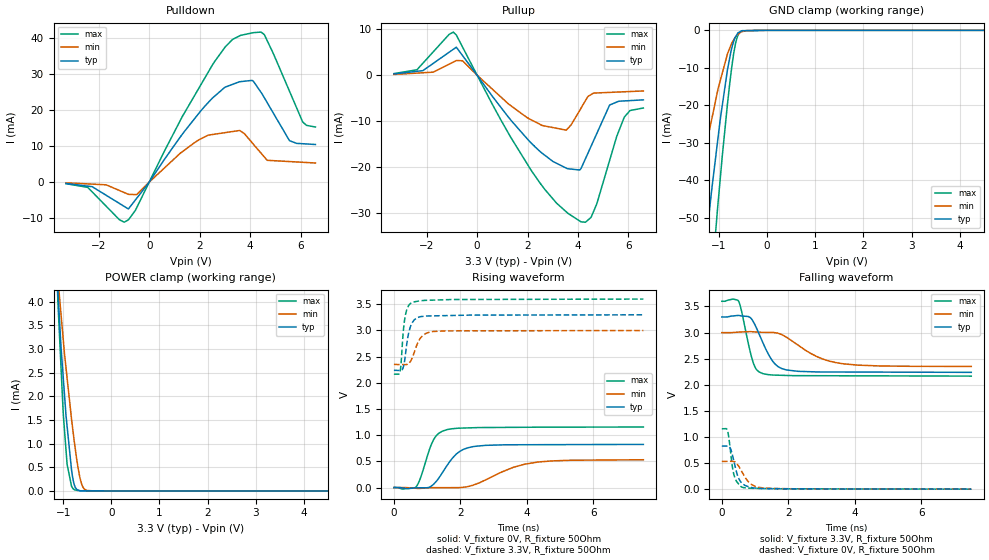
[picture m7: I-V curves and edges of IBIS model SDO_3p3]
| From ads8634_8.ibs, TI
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|   SDO_3p3  3.3V digital 3-state Model
[Model] SDO_3p3  | 3.3V digital 3-state
Model_type 3-state
Polarity   Non-Inverting
Vmeas = 1.65
Vref = 1.65
Cref = 15pF
Rref = 50
|   typ   min   max
|   (nom PVT)   (Fast PVT)   (slow PVT)
|BUFFER OUTPUT TURNED HIGH
|C_comp from L-C Tank method(L=1nH)
|Resonant Frequency(Hz)   4.38G   4.81G   3.96G
|C_comp   1.32459E-12   1.09668E-12   1.61466E-12
|BUFFER OUTPUT LOW
|C_comp from L-C Tank method(L=1nH)
|Resonant Frequency(Hz)   4.29G   4.70G   3.95G
|C_comp   1.38064E-12   1.14552E-12   1.62211E-12
|BUFFER HIGH Z STATE
|C_comp from L-C Tank method(L=1nH)
|Resonant Frequency(Hz)   4.04G   4.41G   3.82G
C_comp   1.55626E-12   1.30641E-12   1.73813E-12
| Where   nom PVT is  Nominal Process, 3.3V, 25C
|   Fast PVT is Strong Process, 3.6V, -40C
|   Slow PVT is Weak Process, 3.0V, 85C
|C_comp - from L-C Tank method, L = 1nH, peak frequency
[Voltage Range]   3.3   3   3.6
[Temperature Range]   27   125   -40
[Pullup Reference]   3.3   3   3.6
[Pulldown Reference]   0   0   0
[Power Clamp Reference]   3.3   3   3.6
[GND Clamp Reference]   0   0   0
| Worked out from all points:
|   slope of the pulldown table from 0 to 0.495 V, typ, clamps not added: 95.7 ohm
|   slope of the pullup table from 0 to 0.495 V, typ, clamps not added: 131 ohm
|   GND clamp passes 1 mA (typ) near -0.62 V on its own axis
|   POWER clamp passes 1 mA (typ) near -0.88 V on its own axis
|   falling waveform, V_fixture 3.3V, R_fixture 50Ohm: 20-80 % time 490ps typ, 1.06ns min, 304ps max; typ from 3.3 V to 2.24 V
|   rising waveform, V_fixture 0V, R_fixture 50Ohm: 20-80 % time 585ps typ, 1.19ns min, 379ps max; typ from 0.002 V to 0.825 V
|   rising waveform, V_fixture 3.3V, R_fixture 50Ohm: 20-80 % time 178ps typ, 264ps min, 129ps max; typ from 2.24 V to 3.3 V
|   falling waveform, V_fixture 0V, R_fixture 50Ohm: 20-80 % time 225ps typ, 337ps min, 161ps max; typ from 0.825 V to 0.002 V
[Pulldown]
|   Voltage   I(typ)   I(min)   I(max)
-3.3V     -389.4uA   -204.7uA   -455.8uA
-2.443V   -1.123mA   -506.1uA   -1.449mA
-1.18V    -5.928mA   -2.343mA   -10.44mA
-825.7mV  -7.447mA   -3.402mA   -10.47mA
-499.9mV  -4.521mA   -3.471mA   -7.151mA
2.512V    23.31mA    13.18mA    32.52mA
3.623V    27.83mA    14.13mA    40.65mA
4.119V    27.98mA    10.56mA    41.38mA
4.56V     23.41mA    6.987mA    40.87mA
5.563V    11.46mA    5.681mA    25.14mA
6.088V    10.62mA    5.477mA    16.62mA
6.59V     10.41mA    5.281mA    15.26mA
[GND Clamp]
|   Voltage   I(typ)   I(min)   I(max)
-3.3V     -333.7mA   -218.9mA   -423.9mA
-1.593V   -96.69mA   -55.56mA   -138.7mA
-1.503V   -85.34mA   -48.26mA   -123.7mA
-1.25V    -54.2mA    -29.86mA   -82.25mA
-1.149V   -42.23mA   -23.57mA   -66.22mA
-1.037V   -30.41mA   -16.66mA   -48.58mA
-826mV    -10.66mA   -6.382mA   -19.88mA
-750.7mV  -5.602mA   -3.917mA   -11.44mA
-698.7mV  -3.129mA   -2.654mA   -6.526mA
-629.4mV  -1.183mA   -1.372mA   -2.157mA
-517.4mV  -87.12uA   -359.9uA   -137.8uA
6.59V     0A         0A         0A
[Pullup]
|   Voltage   I(typ)   I(min)   I(max)
-3.3V     282.6uA    176.9uA    359.9uA
-2.384V   863.4uA    472.2uA    1.213mA
-946.1mV  5.666mA    2.884mA    9.428mA
-576.3mV  4.279mA    3.161mA    6.135mA
1.311V    -9.614mA   -6.549mA   -13.35mA
2.584V    -17.05mA   -10.97mA   -24.2mA
3.534V    -20.28mA   -11.98mA   -29.82mA
4.12V     -20.32mA   -7.166mA   -32.01mA
4.518V    -15.48mA   -4.214mA   -31.01mA
5.251V    -6.512mA   -3.741mA   -18.62mA
5.834V    -5.602mA   -3.604mA   -9.139mA
6.59V     -5.371mA   -3.425mA   -7.146mA
[POWER Clamp]
|   Voltage   I(typ)   I(min)   I(max)
-3.3V     52.32mA    41.51mA    66.09mA
-1.162V   5.162mA    5.3mA      5.365mA
-1.103V   4.107mA    4.473mA    3.873mA
-1.077V   3.627mA    4.11mA     3.306mA
-1.002V   2.452mA    3.25mA     1.719mA
-918.3mV  1.371mA    2.39mA     566.7uA
-826mV    443.1uA    1.521mA    98.85uA
-762mV    112uA      993.2uA    20.84uA
-645.7mV  3.761uA    253.7uA    927.2nA
-584.5mV  2.735uA    71.72uA    604.3nA
-505.2mV  2.351uA    8.775uA    519.3nA
6.59V     0A         0A         0A
[Ramp]
R_load = 50
|   typ   min   max
dV/dt_r   0.493896/5.81927e-010  0.318267/1.16625e-009  0.693599/3.77324e-010
dV/dt_f   0.636389/4.88374e-010  0.388684/1.04617e-009  0.860088/3.02558e-010
[Falling Waveform]
V_fixture = 3.3V
V_fixture_min = 3V
V_fixture_max = 3.6V
R_fixture = 50Ohm
C_fixture = 0F
|   Time   V(typ)   V(min)   V(max)
0s        3.299V     2.999V     3.6V
504.1ps   3.328V     3.01V      3.601V
939.8ps   3.215V     3.015V     2.432V
1.053ns   3.072V     3.01V      2.283V
1.229ns   2.813V     3.005V     2.215V
1.595ns   2.401V     2.998V     2.185V
1.953ns   2.284V     2.908V     2.179V
2.849ns   2.247V     2.543V     2.174V
3.627ns   2.245V     2.404V     2.173V
7.5ns     2.238V     2.351V     2.166V
[Rising Waveform]
V_fixture = 0V
V_fixture_min = 0V
V_fixture_max = 0V
R_fixture = 50Ohm
C_fixture = 0F
|   Time   V(typ)   V(min)   V(max)
0s        1.562mV    1.115mV    646.9uV
667.2ps   -4.062mV   -13.43mV   15mV
798.6ps   -3.843mV   -14.61mV   183mV
1.185ns   58.39mV    -1.454mV   905mV
1.587ns   412.7mV    -1.243mV   1.105V
1.98ns    690.7mV    -304.9uV   1.135V
2.42ns    786.2mV    55.37mV    1.144V
3.575ns   817.7mV    383.1mV    1.15V
4.328ns   819mV      487.4mV    1.153V
7.5ns     824.7mV    531.6mV    1.157V
[Rising Waveform]
V_fixture = 3.3V
V_fixture_min = 3V
V_fixture_max = 3.6V
R_fixture = 50Ohm
C_fixture = 0F
|   Time   V(typ)   V(min)   V(max)
0s        2.238V     2.351V     2.166V
183.3ps   2.237V     2.349V     2.207V
269.2ps   2.275V     2.348V     2.883V
325.5ps   2.442V     2.348V     3.218V
384.4ps   2.733V     2.351V     3.391V
488.1ps   3.058V     2.402V     3.511V
578.3ps   3.174V     2.523V     3.543V
809.1ps   3.265V     2.864V     3.568V
1.181ns   3.279V     2.981V     3.58V
7.5ns     3.299V     2.999V     3.6V
[Falling Waveform]
|Gnd
V_fixture = 0V
V_fixture_min = 0V
V_fixture_max = 0V
R_fixture = 50Ohm
C_fixture = 0F
|   Time   V(typ)   V(min)   V(max)
0s        824.8mV    532.1mV    1.157V
167.1ps   826.4mV    533.3mV    1.128V
253.3ps   788.7mV    533.8mV    766.3mV
316.9ps   659.5mV    534.3mV    430.5mV
369.5ps   518.4mV    529.3mV    262.9mV
486ps     239.4mV    459.2mV    114.1mV
643.2ps   93.98mV    288.3mV    31.56mV
900.5ps   31.84mV    86.94mV    18.06mV
1.238ns   12.15mV    24.65mV    13.93mV
7.5ns     1.613mV    1.435mV    647.5uV
